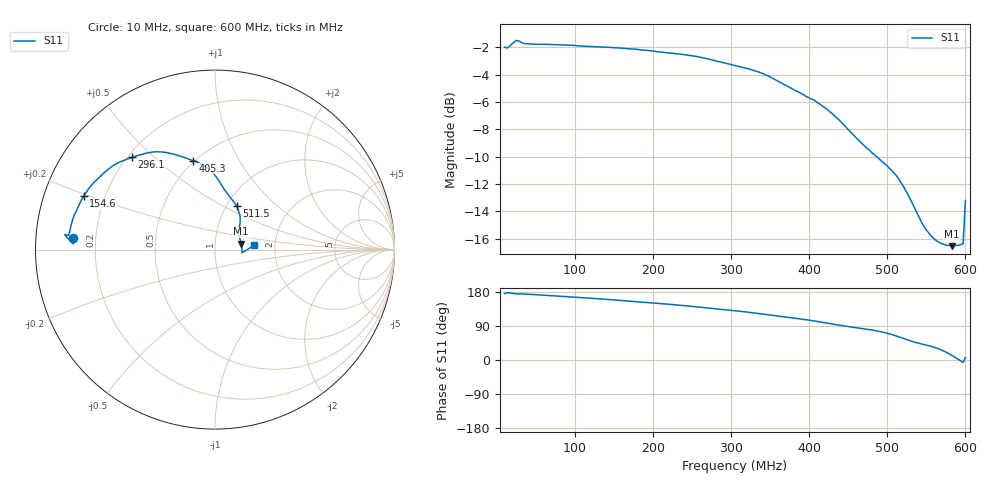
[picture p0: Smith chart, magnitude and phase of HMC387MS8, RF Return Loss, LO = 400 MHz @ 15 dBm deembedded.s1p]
!Hittite Microwave Corporation
!12 Elizabeth Drive
!Chelmsford, MA 01824
!Tel: 978-250-3343
!Fax: 978-250-3373
!Device: HMC387MS8, 450-500 MHz, GaAs MMIC High IP3 Mixer in 8-lead plastic SMT package
!Misc: RF Return Loss, LO = 400 MHz @ 15 dBm, Room
# MHZ S MA R 50
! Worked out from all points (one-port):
!   201 points, 10 MHz to 600 MHz, reference 50 ohm
!   lowest |S11| = -16.5 dB at 582.3 MHz (marker M1), VSWR 1.35, Z = 66.8 + j4.49 ohm
!   |S11| at or under -10 dB: 486.6 MHz to end of sweep
!   S11 on the Smith chart (normalised r, x): 10 MHz: 0.11, +0.04; 154.6 MHz: 0.12, +0.19; 296.1 MHz: 0.22, +0.43; 405.3 MHz: 0.49, +0.66; 511.5 MHz: 1.11, +0.58; 600 MHz: 1.55, +0.08
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10  0.795 175.5
12.95  0.789 177.7
15.9  0.798 177.3
24.75  0.841 174.4
33.6  0.821 174.5
42.45  0.817 173.5
83.75  0.81 168.0
154.55  0.79 157.8
157.5  0.789 157.3
195.85  0.772 151.2
231.25  0.751 145.1
260.75  0.73 139.2
296.15  0.691 131.9
305  0.681 130.0
340.4  0.637 121.1
355.15  0.608 117.0
378.75  0.559 110.9
405.3  0.511 103.7
428.9  0.456 95.3
452.5  0.391 87.5
511.5  0.27 63.5
526.25  0.231 52.8
543.95  0.182 42.3
555.75  0.163 36.2
567.55  0.153 27.9
582.3  0.149 12.7
597.05  0.152 -6.7
600  0.219 6.2
